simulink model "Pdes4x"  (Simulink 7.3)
settings: Solver=ode45  StartTime=0.0  StopTime=10.0  RelTol=1e-3
undefined symbols (not defined in the file or in its folder): Avp, Bvp, Cvp, Dvp

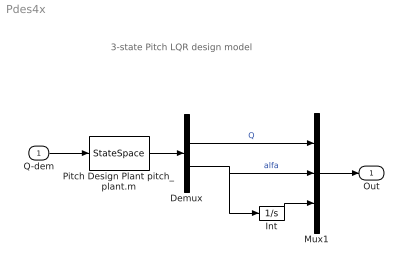
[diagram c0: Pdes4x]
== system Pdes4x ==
  note: 3-state Pitch LQR design model
  Q-dem : Inport  OutDataType=sfix(16)  OutScaling=2^0
  Demux : Demux  Outputs=2
  Int : Integrator
  Mux1 : Mux  Inputs=3
  Pitch Design Plant pitch_plant.m : StateSpace  A=Avp  B=Bvp  C=Cvp  D=Dvp
  Out : Outport  OutDataType=sfix(16)  OutScaling=2^0
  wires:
  Q-dem/1 -> Pitch Design Plant pitch_plant.m/1
  Pitch Design Plant pitch_plant.m/1 -> Demux/1
  Demux/2 -> Int/1, Mux1/2  "alfa"
  Demux/1 -> Mux1/1  "Q"
  Int/1 -> Mux1/3
  Mux1/1 -> Out/1
